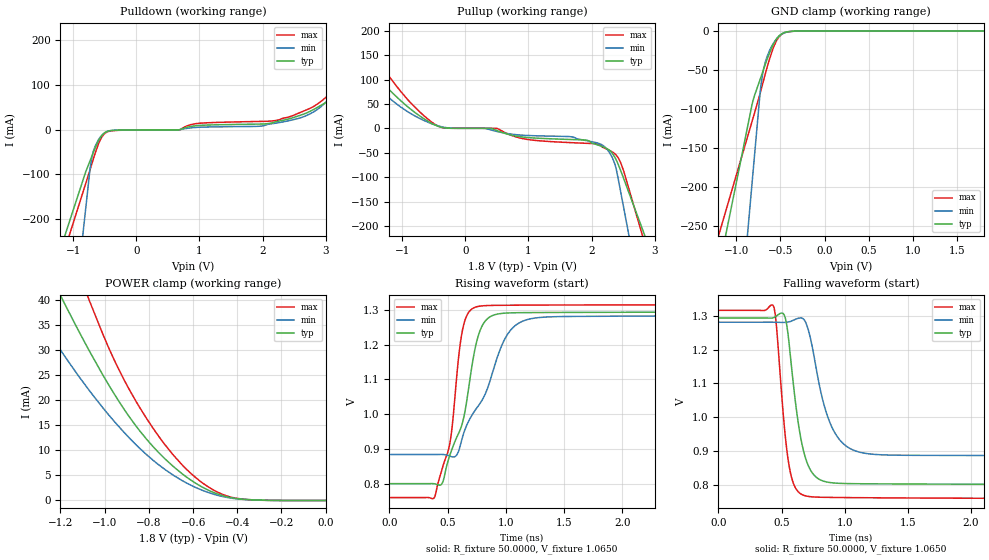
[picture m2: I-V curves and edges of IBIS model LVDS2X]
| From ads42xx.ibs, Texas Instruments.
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|   Model LVDS2X
[Model]  LVDS2X
Model_type 3-state
Polarity   Non-Inverting
Enable   Active-Low
Vmeas =   1.065V
Cref =   5.0000pF
Rref = 50.0000
Vref =   1.065V
C_comp   2.2000pF   2.0000pF   2.4000pF
[Temperature Range]   25.0000   0.1250k   -40.0000
[Voltage Range]   1.8000V   1.7000V   1.9000V
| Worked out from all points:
|   slope of the pulldown table from 0 to 0.27 V, typ, clamps not added: 2.03 kohm
|   slope of the pullup table from 0 to 0.27 V, typ, clamps not added: 19.8 kohm
|   GND clamp passes 1 mA (typ) near -0.42 V on its own axis
|   POWER clamp passes 1 mA (typ) near -0.47 V on its own axis
|   rising waveform, R_fixture 50.0000, V_fixture 1.0650: 20-80 % time 203ps typ, 318ps min, 129ps max; typ from 0.8 V to 1.29 V
|   falling waveform, R_fixture 50.0000, V_fixture 1.0650: 20-80 % time 109ps typ, 159ps min, 80.2ps max; typ from 1.29 V to 0.8 V
[Pulldown]
|Voltage   I(typ)   I(min)   I(max)
-1.8V     -527.4mA   -1.476A    -567.3mA
-800mV    -94.35mA   -176.6mA   -120.5mA
-730mV    -69.23mA   -85.64mA   -89.18mA
-680mV    -51.16mA   -48.73mA   -66mA
-570mV    -17.91mA   -16.81mA   -22.99mA
-460mV    -3.786mA   -3.953mA   -5.011mA
2.17V     15.92mA    13.84mA    19.94mA
2.67V     36mA       30.22mA    42.95mA
2.93V     55.03mA    52.16mA    64mA
3.09V     67.74mA    76.4mA     82.89mA
3.28V     89.19mA    146.6mA    104.4mA
3.6V      150.9mA    277.1mA    138.3mA
[Pullup]
|Voltage   I(typ)   I(min)   I(max)
-1.8V     164.1mA    205.8mA    207.3mA
-1.4V     106.3mA    88.37mA    139.5mA
-910mV    44.17mA    34.17mA    58.83mA
-360mV    1.923mA    2.993mA    1.745mA
490mV     -3.746mA   -5.898mA   297.4uA
970mV     -18.36mA   -14.27mA   -22.23mA
1.91V     -23.88mA   -24.71mA   -30.39mA
2.14V     -35.72mA   -31.99mA   -33.78mA
2.25V     -41.72mA   -43.27mA   -42.9mA
2.37V     -59.27mA   -73.32mA   -52.09mA
2.51V     -103.2mA   -163.4mA   -87.7mA
3.6V      -484.1mA   -908.6mA   -573.5mA
[GND_clamp]
|Voltage   I(typ)   I(min)   I(max)
-1.8V     -644.2mA   -1.444A    -493.9mA
-820mV    -93.96mA   -194.4mA   -115.6mA
-730mV    -62.28mA   -79.59mA   -80.23mA
-720mV    -58.98mA   -69.41mA   -75.99mA
-700mV    -52.31mA   -54.38mA   -67.41mA
-670mV    -42.41mA   -39.65mA   -54.64mA
-620mV    -27.2mA    -24.38mA   -34.87mA
-550mV    -11.15mA   -11.01mA   -13.8mA
-490mV    -3.867mA   -4.474mA   -4.534mA
-420mV    -941.3uA   -1.223mA   -1.169mA
-290mV    -42.52uA   -65.45uA   -73.57uA
1.8V      5.758nA    683.2nA    1.459nA
[POWER_clamp]
|Voltage   I(typ)   I(min)   I(max)
-1.8V     132.7mA    318.5mA    134.1mA
-1.32V    51.78mA    38.91mA    70.46mA
-1.26V    46.2mA     34.09mA    62.77mA
-1.18V    39.07mA    28.66mA    52.85mA
-1.07V    29.83mA    21.92mA    39.87mA
-940mV    20.04mA    14.91mA    26.44mA
-840mV    13.79mA    10.33mA    18.41mA
-730mV    8.407mA    6.259mA    11.26mA
-590mV    3.479mA    2.626mA    4.624mA
-490mV    1.299mA    1.039mA    1.675mA
-410mV    423.1uA    368.9uA    490.9uA
0V        5.758nA    60.92nA    1.932nA
[Ramp]
| variable   typ   min   max
dV/dt_r  0.7029/0.1123n   0.6931/0.1790n   0.7073/81.7215p
dV/dt_f  0.5104/0.1586n   0.4630/0.2633n   0.5449/0.1111n
R_load = 1.0000k
[Rising Waveform]
R_fixture= 50.0000
V_fixture= 1.0650
V_fixture_min= 1.1050
V_fixture_max= 1.0450
|time   V(typ)   V(min)   V(max)
0s        799.7mV    883.7mV    759.6mV
390ps     799mV      883.7mV    762mV
450ps     798.8mV    883.9mV    839.1mV
520ps     882.5mV    878.9mV    917.3mV
580ps     934.5mV    883.1mV    1.116V
630ps     978.2mV    936.3mV    1.246V
770ps     1.233V     1.027V     1.311V
1.02ns    1.291V     1.232V     1.313V
1.3ns     1.293V     1.278V     1.314V
10ns      1.294V     1.287V     1.314V
[Falling Waveform]
R_fixture= 50.0000
V_fixture= 1.0650
V_fixture_min= 1.1050
V_fixture_max= 1.0450
|time   V(typ)   V(min)   V(max)
0s        1.294V     1.281V     1.316V
440ps     1.295V     1.281V     1.325V
520ps     1.303V     1.281V     977.3mV
560ps     1.215V     1.282V     853.4mV
640ps     962.3mV    1.294V     775.5mV
710ps     856.8mV    1.26V      764.9mV
820ps     811.7mV    1.059V     762.3mV
900ps     805.2mV    968.6mV    761.8mV
1.2ns     802.2mV    890.7mV    760.9mV
10ns      799.7mV    886.2mV    758.3mV
